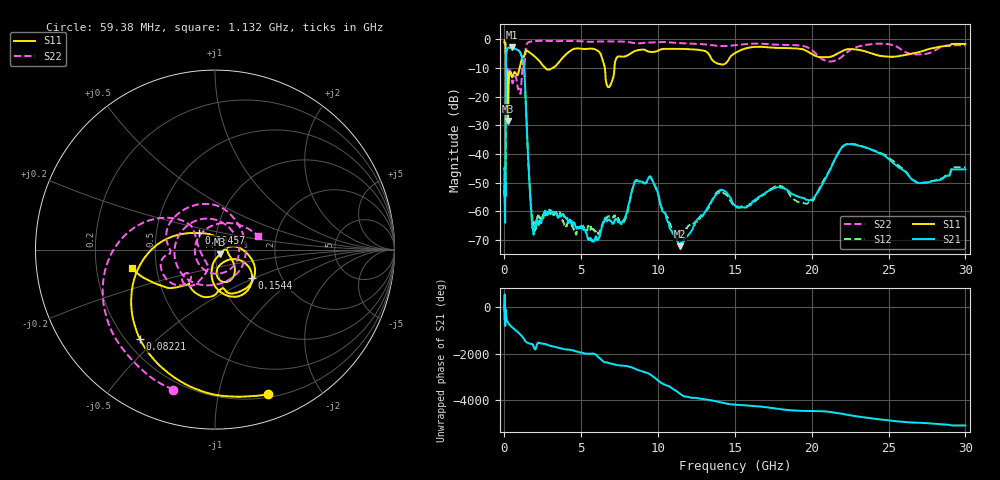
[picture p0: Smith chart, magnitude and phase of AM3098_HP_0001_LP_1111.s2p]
! Date/Time: Thu, Feb 28, 2019 8:32 AM
! Network Analyzer: Agilent Technologies E8364B Rev: A.07.50.67
! Sweep from 0.010 to 30.000 GHz, 1601 Points, Sweep Type: LOG
! Power Supply: 5.023 V, 0.002 A
# Hz S DB R 50
!freq MagS11 AngS11 MagS21 AngS21 MagS12 AngS12 MagS22 AngS22
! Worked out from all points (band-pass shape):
!   1601 points, 10 MHz to 30 GHz, reference 50 ohm
!   highest |S21| = -2.76 dB at 498 MHz (marker M1); lowest = -72.2 dB at 11.42 GHz (marker M2)
!   |S21| within 3 dB of the highest: 106.1 MHz to 1.113 GHz (1.007 GHz wide, 165 % of centre)
!   lowest |S11| = -28.5 dB at 231.6 MHz (marker M3), VSWR 1.08, Z = 52.8 - j2.73 ohm
!   |S11| at or under -10 dB: 91.07 MHz to 973.5 MHz (882.4 MHz wide, 166 % of centre); 2.668 GHz to 3.125 GHz (456.6 MHz wide, 15.8 % of centre); 6.53 GHz to 7.158 GHz (627.5 MHz wide, 9.17 % of centre)
!   |S22| runs from -22.2 to -0.5 dB; largest |S21 - S12| = 0.011
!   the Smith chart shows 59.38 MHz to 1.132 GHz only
!   S11 on the Smith chart (normalised r, x): 59.38 MHz: 0.23, -1.41; 82.21 MHz: 0.26, -0.44; 94.57 MHz: 0.82, +0.15; 154.4 MHz: 1.43, -0.48; 1.132 GHz: 0.36, -0.10
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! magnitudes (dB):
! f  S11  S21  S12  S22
! 10 MHz  -0.3  -45.2  -45.8  -0.6
! 38.04 MHz  -0.5  -58.6  -61.3  -1.1
! 59.38 MHz  -1.3  -53.0  -54.7  -1.8
! 82.21 MHz  -3.7  -33.4  -33.5  -4.1
! 94.57 MHz  -17.8  -11.2  -11.2  -20.6
! 144.7 MHz  -14.5  -3.5  -3.5  -12.8
! 154.4 MHz  -11.7  -3.4  -3.4  -11.2
! 231.6 MHz  -28.5  -2.9  -2.9  -11.9
! 308.1 MHz  -12.4  -2.9  -2.8  -11.1
! 498 MHz  -13.1  -2.8  -2.7  -14.9
! 550.5 MHz  -12.6  -2.9  -2.9  -15.1
! 1.132 GHz  -6.5  -6.1  -6.1  -12.0
! 1.308 GHz  -5.4  -12.2  -12.1  -8.9
! 1.82 GHz  -5.3  -65.9  -62.3  -0.6
! 2.084 GHz  -6.5  -63.4  -64.9  -0.5
! 7.926 GHz  -5.8  -60.9  -61.7  -0.8
! 9.49 GHz  -4.3  -47.8  -47.9  -1.1
! 11.42 GHz  -3.3  -72.2  -68.1  -1.2
! 14.02 GHz  -8.6  -52.9  -52.6  -2.3
! 19.61 GHz  -3.8  -55.9  -57.3  -2.5
! 22.67 GHz  -3.4  -36.7  -36.5  -3.2
! 30 GHz  -1.5  -45.3  -44.6  -2.0
